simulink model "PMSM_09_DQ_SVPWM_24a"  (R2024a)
settings: Solver=ode45  StartTime=0.0  StopTime=0.1  MaxStep=1e-6  RelTol=1e-6  AbsTol=1e-6  EnableMultiTasking=on
undefined symbols (not defined in the file): by, established, Flux, linkage, magnets, V
libraries: spsIGBTDiodeLib x6, spsCurrentMeasurementLib x3, slpidlib x2, spsDCVoltageSourceLib x1, spsPermanentMagnetSynchronousMachineLib x1, simulink x1, spspowerguiLib x1

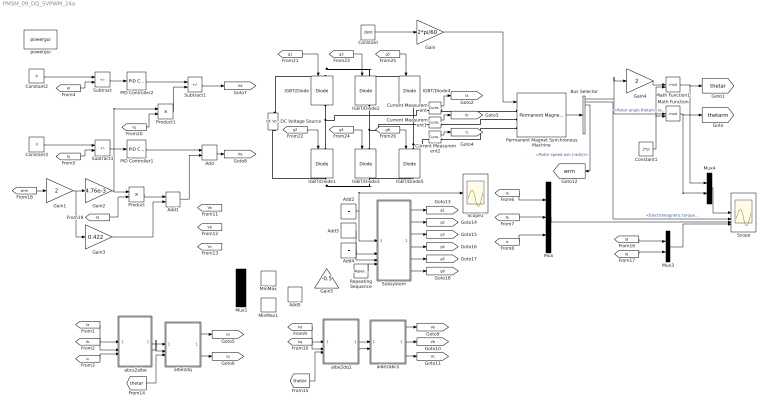
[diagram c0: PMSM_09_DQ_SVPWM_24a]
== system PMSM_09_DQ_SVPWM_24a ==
  Add{,1..5} (6 alike) : Sum
  Bus Selector : BusSelector  OutputSignals=Rotor angle thetam (rad),Electromagnetic torque Te (N*m),Rotor speed wm (rad/s)
  Constant : Constant  Value=2600
  Constant1 : Constant  Value=2*pi
  Constant2 : Constant  Value=0
  Constant3 : Constant  Value=3
  Current Measurement : spsCurrentMeasurementLib/Current Measurement  PhasorSimulation=off  OutputType=Complex  PSBequivalent=0
  Current Measurement1 : spsCurrentMeasurementLib/Current Measurement  PhasorSimulation=off  OutputType=Complex  PSBequivalent=0
  Current Measurement2 : spsCurrentMeasurementLib/Current Measurement  PhasorSimulation=off  OutputType=Complex  PSBequivalent=0
  DC Voltage Source : spsDCVoltageSourceLib/DC Voltage Source  Amplitude=400  Measurements=None
  Gain : Gain  Gain=2*pi/60
  Gain1 : Gain  Gain=2
  Gain2 : Gain  Gain=4.76e-3
  Gain3 : Gain  Gain=0.422
  Gain4 : Gain  Gain=2
  Gain5 : Gain  Gain=-0.5
  IGBT/Diode{,1..5} (6 alike) : spsIGBTDiodeLib/IGBT//Diode  Ron=1e-3  Rs=1e5  Cs=inf  Measurements=on
  Math Function : Math  Operator=mod  SignedPower=on
  Math Function1 : Math  Operator=mod  SignedPower=on
  MinMax : MinMax
  MinMax1 : MinMax  Function=max
  Mux : Mux  Inputs=3
  Mux1 : Mux  Inputs=3
  Mux3 : Mux  Inputs=2
  Mux4 : Mux  Inputs=2
  PID Controller1 : slpidlib/PID Controller  Controller=PI  Form=Parallel  TimeDomain=Continuous-time  UseExternalTs=off  SampleTime=1  IntegratorMethod=Forward Euler  FilterMethod=Forward Euler  ControllerParametersSource=internal  P=14.95  I=1328.9  UseKiTs=off  D=0  UseExternalDerivativeSource=off  N=100  UseFilter=on  TunerSelectOption=Transfer Function Based (PID Tuner App)  InitialConditionSource=internal  InitialConditionForIntegrator=0  InitialConditionForFilter=0  DifferentiatorICPrevScaledInput=0  ExternalReset=none  TrackingMode=off  Kt=1  LimitOutput=off  SatLimitsSource=internal  UpperSaturationLimit=inf  LowerSaturationLimit=-inf  LinearizeAsGain=on  AntiWindupMode=none  Kb=1  LimitIntegrator=off  UpperIntegratorSaturationLimit=inf  LowerIntegratorSaturationLimit=-inf  POutMin=[]  POutMax=[]  IOutMin=[]  IOutMax=[]  DOutMin=[]  DOutMax=[]  NOutMin=[]  NOutMax=[]  SumOutMin=[]  SumOutMax=[]  SaturationOutMin=[]  SaturationOutMax=[]  PParamMin=[]  PParamMax=[]  IParamMin=[]  IParamMax=[]  DParamMin=[]  DParamMax=[]  NParamMin=[]  NParamMax=[]  KbParamMin=[]  KbParamMax=[]  KtParamMin=[]  KtParamMax=[]  KbOutMin=[]  KbOutMax=[]  KtOutMin=[]  KtOutMax=[]  IntegratorOutMin=[]  IntegratorOutMax=[]  FilterOutMin=[]  FilterOutMax=[]  SumI1OutMin=[]  SumI1OutMax=[]  SumI2OutMin=[]  SumI2OutMax=[]  SumI3OutMin=[]  SumI3OutMax=[]  SumI4OutMin=[]  SumI4OutMax=[]  SumDOutMin=[]  SumDOutMax=[]  DifferentiatorOutMin=[]  DifferentiatorOutMax=[]  FilterDiffOutCoefMin=[]  FilterDiffOutCoefMax=[]  ReciprocalOutMin=[]  ReciprocalOutMax=[]  SumDenOutMin=[]  SumDenOutMax=[]  SumNumOutMin=[]  SumNumOutMax=[]  DivideOutMin=[]  DivideOutMax=[]  UdiffTsProdOutMin=[]  UdiffTsProdOutMax=[]  NTsProdOutMin=[]  NTsProdOutMax=[]  UintegralTsProdOutMin=[]  UintegralTsProdOutMax=[]  UngainTsProdOutMin=[]  UngainTsProdOutMax=[]  ClampingZeroOutDataTypeStr=Inherit: Inherit via back propagation  ClampingZeroOutMin=[]  ClampingZeroOutMax=[]  FilterDenConstantOutDataTypeStr=Inherit: Inherit via back propagation  FilterDenConstantOutMin=[]  FilterDenConstantOutMax=[]  PCopyOutDataTypeStr=Inherit: Inherit via back propagation  PCopyOutMin=[]  PCopyOutMax=[]  NCopyOutDataTypeStr=Inherit: Inherit via back propagation  NCopyOutMin=[]  NCopyOutMax=[]  IntegratorContinuousStateAttributes=''  IntegratorStateMustResolveToSignalObject=off  IntegratorRTWStateStorageClass=Auto  FilterContinuousStateAttributes=''  FilterStateMustResolveToSignalObject=off  FilterRTWStateStorageClass=Auto  ParallelPVariant=InternalParameters  IdealPVariant=Disabled  IVariant=InternalParameters  DVariant=Disabled  IntegratorVariant=Continuous  SatVariant=Disabled  AWVariant=Passthrough  PCopyVariant=Disabled  TRVariant=Disabled  FdbkBlocksVariant=Forward  IdealPFdbkVariant=Disabled  SatFdbkVariant=Disabled  DerivativeFilterVariant=Disabled  NVariant=Disabled  NCopyVariant=Disabled_SignalSpec  FilterICVariant=Disabled  IntegratorICVariant=InternalICs  ExternalResetVariant=Disabled  TRSumVariant=Passthrough  SumFdbkVariant=Disabled  SumVariant=Sum_PI  TsampFilterVariant=InternalTs  TsampNgainVariant=Passthrough  TsampIntegralVariant=Disabled_SignalSpec  ExternalSaturationOutDataTypeStr=Inherit: Same as second input  DerivativeSourceVariant=Disabled
  PID Controller2 : slpidlib/PID Controller  Controller=PI  Form=Parallel  TimeDomain=Continuous-time  UseExternalTs=off  SampleTime=1  IntegratorMethod=Forward Euler  FilterMethod=Forward Euler  ControllerParametersSource=internal  P=14.95  I=1328.9  UseKiTs=off  D=0  UseExternalDerivativeSource=off  N=100  UseFilter=on  TunerSelectOption=Transfer Function Based (PID Tuner App)  InitialConditionSource=internal  InitialConditionForIntegrator=0  InitialConditionForFilter=0  DifferentiatorICPrevScaledInput=0  ExternalReset=none  TrackingMode=off  Kt=1  LimitOutput=off  SatLimitsSource=internal  UpperSaturationLimit=inf  LowerSaturationLimit=-inf  LinearizeAsGain=on  AntiWindupMode=none  Kb=1  LimitIntegrator=off  UpperIntegratorSaturationLimit=inf  LowerIntegratorSaturationLimit=-inf  POutMin=[]  POutMax=[]  IOutMin=[]  IOutMax=[]  DOutMin=[]  DOutMax=[]  NOutMin=[]  NOutMax=[]  SumOutMin=[]  SumOutMax=[]  SaturationOutMin=[]  SaturationOutMax=[]  PParamMin=[]  PParamMax=[]  IParamMin=[]  IParamMax=[]  DParamMin=[]  DParamMax=[]  NParamMin=[]  NParamMax=[]  KbParamMin=[]  KbParamMax=[]  KtParamMin=[]  KtParamMax=[]  KbOutMin=[]  KbOutMax=[]  KtOutMin=[]  KtOutMax=[]  IntegratorOutMin=[]  IntegratorOutMax=[]  FilterOutMin=[]  FilterOutMax=[]  SumI1OutMin=[]  SumI1OutMax=[]  SumI2OutMin=[]  SumI2OutMax=[]  SumI3OutMin=[]  SumI3OutMax=[]  SumI4OutMin=[]  SumI4OutMax=[]  SumDOutMin=[]  SumDOutMax=[]  DifferentiatorOutMin=[]  DifferentiatorOutMax=[]  FilterDiffOutCoefMin=[]  FilterDiffOutCoefMax=[]  ReciprocalOutMin=[]  ReciprocalOutMax=[]  SumDenOutMin=[]  SumDenOutMax=[]  SumNumOutMin=[]  SumNumOutMax=[]  DivideOutMin=[]  DivideOutMax=[]  UdiffTsProdOutMin=[]  UdiffTsProdOutMax=[]  NTsProdOutMin=[]  NTsProdOutMax=[]  UintegralTsProdOutMin=[]  UintegralTsProdOutMax=[]  UngainTsProdOutMin=[]  UngainTsProdOutMax=[]  ClampingZeroOutDataTypeStr=Inherit: Inherit via back propagation  ClampingZeroOutMin=[]  ClampingZeroOutMax=[]  FilterDenConstantOutDataTypeStr=Inherit: Inherit via back propagation  FilterDenConstantOutMin=[]  FilterDenConstantOutMax=[]  PCopyOutDataTypeStr=Inherit: Inherit via back propagation  PCopyOutMin=[]  PCopyOutMax=[]  NCopyOutDataTypeStr=Inherit: Inherit via back propagation  NCopyOutMin=[]  NCopyOutMax=[]  IntegratorContinuousStateAttributes=''  IntegratorStateMustResolveToSignalObject=off  IntegratorRTWStateStorageClass=Auto  FilterContinuousStateAttributes=''  FilterStateMustResolveToSignalObject=off  FilterRTWStateStorageClass=Auto  ParallelPVariant=InternalParameters  IdealPVariant=Disabled  IVariant=InternalParameters  DVariant=Disabled  IntegratorVariant=Continuous  SatVariant=Disabled  AWVariant=Passthrough  PCopyVariant=Disabled  TRVariant=Disabled  FdbkBlocksVariant=Forward  IdealPFdbkVariant=Disabled  SatFdbkVariant=Disabled  DerivativeFilterVariant=Disabled  NVariant=Disabled  NCopyVariant=Disabled_SignalSpec  FilterICVariant=Disabled  IntegratorICVariant=InternalICs  ExternalResetVariant=Disabled  TRSumVariant=Passthrough  SumFdbkVariant=Disabled  SumVariant=Sum_PI  TsampFilterVariant=InternalTs  TsampNgainVariant=Passthrough  TsampIntegralVariant=Disabled_SignalSpec  ExternalSaturationOutDataTypeStr=Inherit: Same as second input  DerivativeSourceVariant=Disabled
  Permanent Magnet Synchronous Machine : spsPermanentMagnetSynchronousMachineLib/Permanent Magnet Synchronous Machine  NbPhases=3  FluxDistribution=Sinusoidal  RotorType=Round  MechanicalLoad=Speed w  PresetModel=No  ShowDetailedParameters=on  MeasurementBus=off  Resistance=0.423  Inductance=8.5e-3  dqInductances=[8.5e-3,8.5e-3]  La=0.00476  MachineConstant=Flux linkage established by magnets (V.s)  Flux=0.422  VoltageCst=153.0847  TorqueCst=1.266  Flat=120  Mechanical=[0.03 0.04 4 0]  PolePairs=2  InitialConditions=[0,0, 0,0]  InitialConditions5ph=[0 0 0 0 0 0]  RefAngle=Aligned with phase A axis (original Park)  IterativeDiscreteModel=Trapezoidal non iterative  TsBlock=-1  TsPowergui=0
  Product : Product
  Product1 : Product
  Repeating Sequence : simulink/Sources/Repeating Sequence  rep_seq_t=[0 0.00005 0.0001]  rep_seq_y=[-200 200 -200]
  Scope : Scope  NumInputPorts=4
  Scope1 : Scope
  Subsystem : Subsystem
  Subtract : Sum  Inputs=+-
  Subtract1 : Sum  Inputs=+-
  Subtract3 : Sum  Inputs=+-
  abcs2albe : Subsystem
  albe2abcs : Subsystem
  albe2dq : Subsystem
  albe2dq1 : Subsystem
  powergui : spspowerguiLib/powergui  Priority=1  SimulationMode=Continuous  SampleTime=50e-6  frequency=60  Iterations=50  frequencyindice=0  Pbase=100e6  ErrMax=1e-4  UnitsV=kV  UnitsW=MW  buscounter=0  FunctionMessages=off  echomessages=off  EnableUseOfTLC=off  CurrentSourceSwitches=off  DisableSnubberDevices=on  DisableRonSwitches=on  DisableVfSwitches=on  DisplayEquations=off  AutomaticDiscreteSolvers=off  SolverType=Tustin  Interpol=off  ExternalGateDelay=off  methode=off  Ts=0  x0status=blocks  SPID=on  SwTol=0  HookPort=off  NonlinearTolerance=1e-4  nMaxIteration=100  ContinueOnMaxIteration=off  RestoreLinks=warning  ResistiveCurrentMeasurement=off  Frange=[0:2:500]  Ylog=off  Xlog=on  ShowGrid=off  save=off  variable=ZData  structure=0  ZoomFFT=off  StartTime=0.0  cycles=1  DisplayStyle=1  fundamental=60  FreqAxis=off  MaxFrequency=1000  frequencyindicesteady=1  RmsSteady=1  display=off
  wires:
  Gain/1 -> Permanent Magnet Synchronous Machine/1
  Constant/1 -> Gain/1
  Subtract/1 -> PID Controller2/1
  Permanent Magnet Synchronous Machine/1 -> Bus Selector/1
  Mux/1 -> Scope/3
  Bus Selector/2 -> Scope/2  "<Electromagnetic torque Te (N*m)>"
  Bus Selector/1 -> Gain4/1, Math Function/1  "<Rotor angle thetam (rad)>"
  Constant1/1 -> Math Function1/2, Math Function/2
  Math Function/1 -> Mux4/2, [thetarm]
  Gain4/1 -> Math Function1/1
  Math Function1/1 -> Mux4/1, [thetar]
  Subtract3/1 -> PID Controller1/1
  [Id] -> Subtract/2
  [Iq] -> Subtract3/2
  [Ia] -> Mux/1
  [Ib] -> Mux/2
  [Ic] -> Mux/3
  Mux3/1 -> Scope/4
  [Id] -> Mux3/1
  [Iq] -> Mux3/2
  Mux4/1 -> Scope/1
  albe2dq1/1(alpha) -> albe2abcs/1(alpha)
  albe2dq1/2(beta) -> albe2abcs/2(beta)
  albe2abcs/1(as) -> [Va]
  albe2abcs/2(bs) -> [Vb]
  albe2abcs/3(cs) -> [Vc]
  [Ia] -> abcs2albe/1(as)
  [Ib] -> abcs2albe/2(bs)
  [Ic] -> abcs2albe/3(cs)
  Bus Selector/3 -> [wrm]  "<Rotor speed wm (rad/s)>"
  abcs2albe/1(alpha) -> albe2dq/1(alpha)
  abcs2albe/2(beta) -> albe2dq/2(beta)
  albe2dq/1(d) -> [Id]
  albe2dq/2(q) -> [Iq]
  [thetar] -> albe2dq/3(thetar)
  [Vq] -> albe2dq1/2(q)
  [Vd] -> albe2dq1/1(d)
  [thetar] -> albe2dq1/3(thetar)
  Constant3/1 -> Subtract3/1
  PID Controller1/1 -> Add/1
  Add/1 -> [Vq]
  [wrm] -> Gain1/1
  Gain1/1 -> Gain3/1, Gain2/1
  Gain2/1 -> Product1/1, Product/1
  [Id] -> Product/2
  Product/1 -> Add1/1
  Gain3/1 -> Add1/2
  Add1/1 -> Add/2
  PID Controller2/1 -> Subtract1/1
  Subtract1/1 -> [Vd]
  Product1/1 -> Subtract1/2
  [Iq] -> Product1/2
  [g1] -> IGBT/Diode/1
  [g2] -> IGBT/Diode1/1
  [g3] -> IGBT/Diode2/1
  [g4] -> IGBT/Diode3/1
  [g5] -> IGBT/Diode4/1
  [g6] -> IGBT/Diode5/1
  Current Measurement/1 -> [Ia]
  Current Measurement1/1 -> [Ib]
  Current Measurement2/1 -> [Ic]
  Repeating Sequence/1 -> Subsystem/4(Car)
  Subsystem/1(g1) -> [g1]
  Subsystem/2(g2) -> [g2]
  Subsystem/3(g3) -> [g3]
  Subsystem/4(g4) -> [g4]
  Subsystem/5(g5) -> [g5]
  Subsystem/6(g6) -> [g6]
  Add4/1 -> Subsystem/3(Vcn)
  Add3/1 -> Subsystem/2(Vbn)
  Add2/1 -> Scope1/1, Subsystem/1(Van)
  Constant2/1 -> Subtract/1
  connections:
  IGBT/Diode1/LConn1 -- Current Measurement/LConn1 -- IGBT/Diode/RConn1
  IGBT/Diode3/LConn1 -- Current Measurement1/LConn1 -- IGBT/Diode2/RConn1
  IGBT/Diode5/LConn1 -- Current Measurement2/LConn1 -- IGBT/Diode4/RConn1
  DC Voltage Source/RConn1 -- IGBT/Diode4/LConn1 -- IGBT/Diode2/LConn1 -- IGBT/Diode/LConn1
  IGBT/Diode1/RConn1 -- IGBT/Diode5/RConn1 -- IGBT/Diode3/RConn1 -- DC Voltage Source/LConn1
  Current Measurement2/RConn1 -- Permanent Magnet Synchronous Machine/LConn3
  Current Measurement1/RConn1 -- Permanent Magnet Synchronous Machine/LConn2
  Current Measurement/RConn1 -- Permanent Magnet Synchronous Machine/LConn1

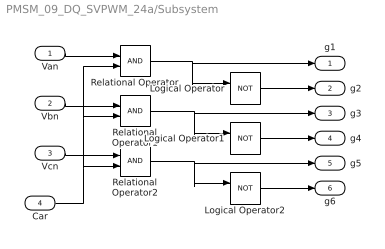
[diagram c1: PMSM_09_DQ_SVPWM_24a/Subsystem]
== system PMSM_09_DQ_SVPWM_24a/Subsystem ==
  Van : Inport
  Vbn : Inport  Port=2
  Vcn : Inport  Port=3
  Car : Inport  Port=4
  Logical Operator : Logic  Operator=NOT  AllPortsSameDT=off  OutDataTypeStr=boolean
  Logical Operator1 : Logic  Operator=NOT  AllPortsSameDT=off  OutDataTypeStr=boolean
  Logical Operator2 : Logic  Operator=NOT  AllPortsSameDT=off  OutDataTypeStr=boolean
  Relational Operator : RelationalOperator  OutDataTypeStr=boolean
  Relational Operator1 : RelationalOperator  OutDataTypeStr=boolean
  Relational Operator2 : RelationalOperator  OutDataTypeStr=boolean
  g1 : Outport
  g2 : Outport  Port=2
  g3 : Outport  Port=3
  g4 : Outport  Port=4
  g5 : Outport  Port=5
  g6 : Outport  Port=6
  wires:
  Relational Operator2/1 -> g5/1, Logical Operator2/1
  Relational Operator1/1 -> g3/1, Logical Operator1/1
  Relational Operator/1 -> g1/1, Logical Operator/1
  Logical Operator2/1 -> g6/1
  Logical Operator1/1 -> g4/1
  Logical Operator/1 -> g2/1
  Car/1 -> Relational Operator/2, Relational Operator1/2, Relational Operator2/2
  Vcn/1 -> Relational Operator2/1
  Vbn/1 -> Relational Operator1/1
  Van/1 -> Relational Operator/1

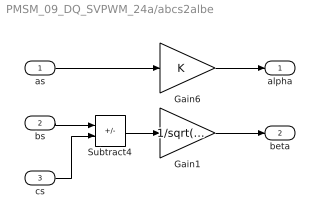
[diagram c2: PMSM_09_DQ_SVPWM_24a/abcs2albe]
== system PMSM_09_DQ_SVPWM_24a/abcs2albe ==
  as : Inport
  bs : Inport  Port=2
  cs : Inport  Port=3
  Gain1 : Gain  Gain=1/sqrt(3)
  Gain6 : Gain
  Subtract4 : Sum  Inputs=+-
  alpha : Outport
  beta : Outport  Port=2
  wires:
  bs/1 -> Subtract4/1
  as/1 -> Gain6/1
  cs/1 -> Subtract4/2
  Gain1/1 -> beta/1
  Subtract4/1 -> Gain1/1
  Gain6/1 -> alpha/1

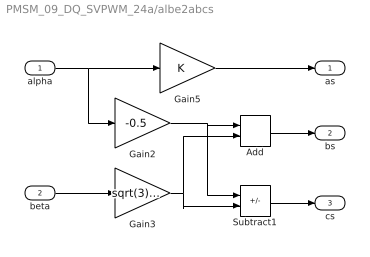
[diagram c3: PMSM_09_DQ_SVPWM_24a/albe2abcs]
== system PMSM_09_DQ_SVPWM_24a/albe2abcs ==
  alpha : Inport
  beta : Inport  Port=2
  Add : Sum
  Gain2 : Gain  Gain=-0.5
  Gain3 : Gain  Gain=sqrt(3)/2
  Gain5 : Gain
  Subtract1 : Sum  Inputs=+-
  as : Outport
  bs : Outport  Port=2
  cs : Outport  Port=3
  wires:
  alpha/1 -> Gain2/1, Gain5/1
  Gain3/1 -> Subtract1/2, Add/2
  Gain2/1 -> Subtract1/1, Add/1
  Add/1 -> bs/1
  Subtract1/1 -> cs/1
  beta/1 -> Gain3/1
  Gain5/1 -> as/1

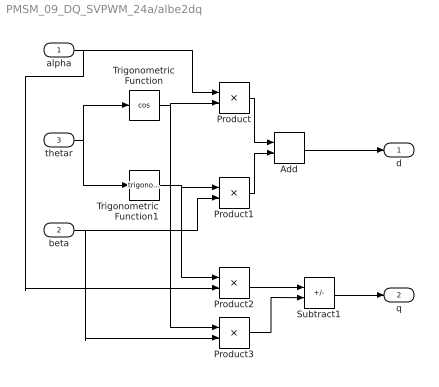
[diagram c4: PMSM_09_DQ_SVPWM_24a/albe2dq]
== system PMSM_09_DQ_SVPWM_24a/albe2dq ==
  alpha : Inport
  beta : Inport  Port=2
  thetar : Inport  Port=3
  Add : Sum
  Product{,1..3} (4 alike) : Product
  Subtract1 : Sum  Inputs=-+
  Trigonometric Function : Trigonometry  Operator=cos
  Trigonometric Function1 : Trigonometry
  d : Outport
  q : Outport  Port=2
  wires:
  thetar/1 -> Trigonometric Function/1, Trigonometric Function1/1
  Trigonometric Function/1 -> Product3/1, Product/2
  Trigonometric Function1/1 -> Product2/1, Product1/1
  beta/1 -> Product3/2, Product1/2
  Product/1 -> Add/1
  Product1/1 -> Add/2
  Add/1 -> d/1
  Subtract1/1 -> q/1
  alpha/1 -> Product/1, Product2/2
  Product2/1 -> Subtract1/1
  Product3/1 -> Subtract1/2

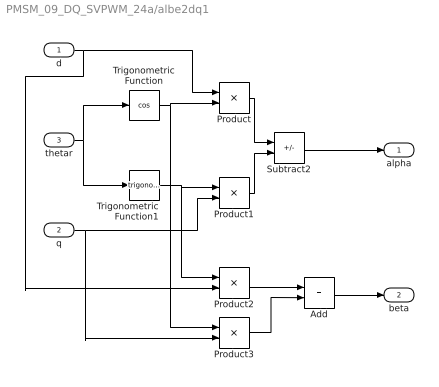
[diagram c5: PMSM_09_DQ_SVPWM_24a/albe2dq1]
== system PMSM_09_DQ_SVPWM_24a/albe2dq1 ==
  d : Inport
  q : Inport  Port=2
  thetar : Inport  Port=3
  Add : Sum
  Product{,1..3} (4 alike) : Product
  Subtract2 : Sum  Inputs=+-
  Trigonometric Function : Trigonometry  Operator=cos
  Trigonometric Function1 : Trigonometry
  alpha : Outport
  beta : Outport  Port=2
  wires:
  Product3/1 -> Add/2
  Product2/1 -> Add/1
  d/1 -> Product2/2, Product/1
  Add/1 -> beta/1
  Subtract2/1 -> alpha/1
  Product1/1 -> Subtract2/2
  Product/1 -> Subtract2/1
  q/1 -> Product1/2, Product3/2
  Trigonometric Function1/1 -> Product1/1, Product2/1
  Trigonometric Function/1 -> Product/2, Product3/1
  thetar/1 -> Trigonometric Function1/1, Trigonometric Function/1
